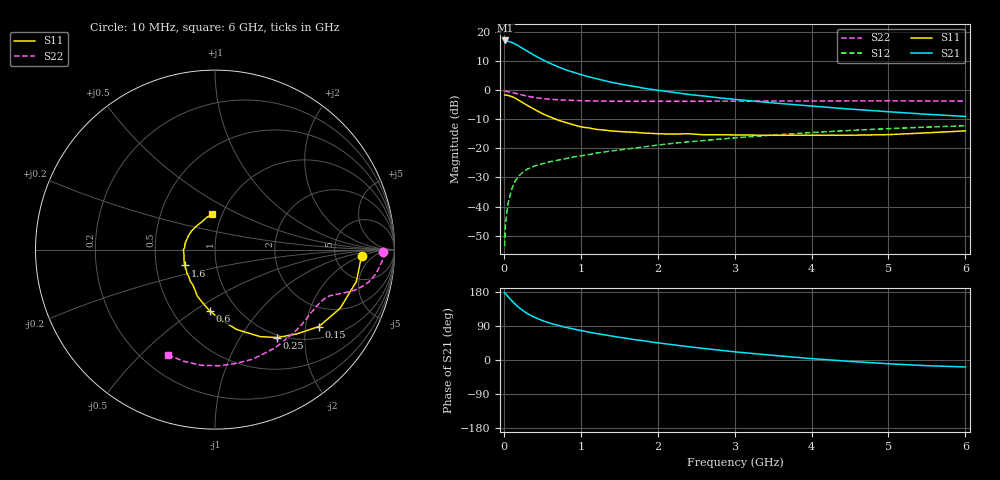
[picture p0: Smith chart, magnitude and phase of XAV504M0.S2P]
! SIEMENS Discrete & RF Semiconductors
! BFY180
! Si NPN RF Bipolar Junction Transistor in MICRO-X
! VCE = 0.5 V  IC = 4 mA
! Common Emitter S-Parameters:  May  1997
# GHz  S  MA  R  50
!  f  S11  S21  S12  S22
! GHz  MAG  ANG  MAG  ANG  MAG  ANG  MAG  ANG
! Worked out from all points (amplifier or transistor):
!   36 points, 10 MHz to 6 GHz, reference 50 ohm
!   highest |S21| = 16.9 dB at 20 MHz (marker M1)
!   |S21| within 3 dB of that: start of sweep to 261.4 MHz
!   unconditionally stable (mu >= 1): start of sweep to 13.74 MHz; 358.4 MHz to end of sweep
!   at 250 MHz: K = 0.75, MSG = 21.1 dB, |S12| = -28.1 dB
!   at 1.4 GHz: K = 2.37, MAG = 5.2 dB, |S12| = -20.9 dB
!   at 6 GHz: K = 3.23, MAG = -6.4 dB, |S12| = -12.3 dB
!   S11 on the Smith chart (normalised r, x): 10 MHz: 9.46, -2.11; 150 MHz: 1.33, -2.38; 250 MHz: 0.96, -1.47; 600 MHz: 0.75, -0.58; 1.6 GHz: 0.70, -0.13; 6 GHz: 0.89, +0.37
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0.01  0.8171 -2.6  6.921 177.8  0.0021 79.6  0.9379 -0.9
0.02  0.8123 -5.2  7.025 175.1  0.0047 85.6  0.9445 -1.8
0.05  0.8072 -12.8  6.819 168.3  0.0107 80.7  0.9307 -4.4
0.1  0.77 -25.2  6.539 157.0  0.0196 73.4  0.9074 -8.5
0.15  0.7203 -36.5  6.096 146.7  0.0278 66.9  0.8757 -11.9
0.2  0.655 -45.8  5.569 137.8  0.0339 61.1  0.8418 -14.3
0.25  0.5999 -54.8  5.074 130.2  0.0392 57.0  0.8107 -16.2
0.3  0.546 -62.6  4.647 123.2  0.0435 53.6  0.7814 -17.5
0.4  0.4614 -74.8  3.882 112.6  0.0497 49.6  0.7408 -19.3
0.5  0.3927 -85.2  3.298 104.2  0.0541 46.9  0.7115 -20.7
0.6  0.3437 -94.8  2.854 97.1  0.0587 45.8  0.691 -21.8
0.7  0.3046 -102.9  2.502 91.7  0.0623 45.0  0.6772 -23.0
0.8  0.2772 -110.9  2.222 86.4  0.0663 45.1  0.6667 -24.4
1.1  0.2236 -127.9  1.68 73.9  0.0775 44.8  0.6492 -28.8
1.4  0.1978 -143.2  1.35 63.3  0.0899 44.4  0.6392 -33.8
1.6  0.1899 -152.2  1.2 57.1  0.0971 44.3  0.6389 -37.3
2.2  0.1745 -173.5  0.91 40.2  0.1212 41.6  0.6368 -48.1
2.8  0.1702 169.6  0.73 26.1  0.1433 38.2  0.6409 -58.7
3.5  0.1668 152.5  0.598 12.3  0.1683 33.5  0.6455 -71.0
4.5  0.167 128.6  0.469 -3.7  0.2019 25.0  0.6475 -88.2
5.5  0.1835 105.6  0.382 -15.0  0.2303 16.3  0.646 -105.6
6  0.1983 95.0  0.351 -18.4  0.2429 11.8  0.6423 -113.8
